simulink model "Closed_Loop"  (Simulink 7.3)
settings: Solver=ode45  StartTime=0.0  StopTime=10.0  RelTol=1e-3
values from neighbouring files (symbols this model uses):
  Acl = [    [closedloop.m]    (also in closedloop_eo.m)
  Bcl = [    [closedloop.m]    (also in closedloop_eo.m)
  Ccl = [    [closedloop.m]    (also in closedloop_eo.m)
  Dcl = [    [closedloop.m]    (also in closedloop_eo.m)

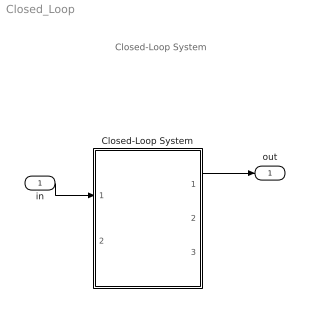
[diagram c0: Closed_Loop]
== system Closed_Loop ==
  note: Closed-Loop System
  in : Inport  OutDataType=sfix(16)  OutScaling=2^0
  Closed-Loop System : Subsystem
  out : Outport  OutDataType=sfix(16)  OutScaling=2^0
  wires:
  in/1 -> Closed-Loop System/1(atti)
  Closed-Loop System/1(attit) -> out/1

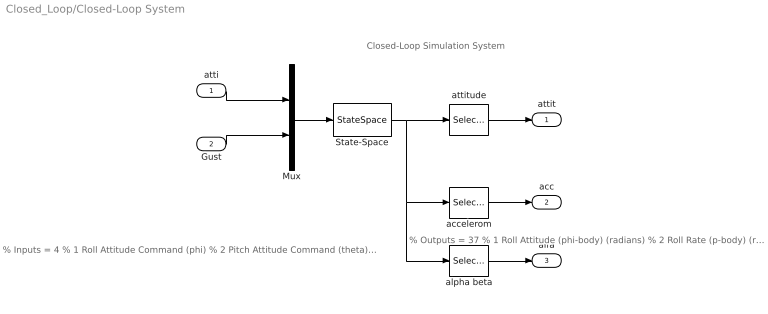
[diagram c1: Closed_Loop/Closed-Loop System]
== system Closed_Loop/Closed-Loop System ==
  note: % Inputs = 4 % 1 Roll Attitude Command (phi) % 2 Pitch Attitude Command (theta) % 3 Yaw Attitude Command (psi) % 4 Wind Gust Velocity (ft/sec)
  note: % Outputs = 37 % 1 Roll Attitude (phi-body) (radians) % 2 Roll Rate (p-body) (rad/sec) % 3 Pitch Attitude (thet-bdy) (radians) % 4 Pitch Rate (q-body) (rad/sec) % 5 Yaw Attitude (psi-body) (radians) % 6 Yaw Rate (r-body) (rad/sec) % 7 Angle of attack, alfa, (radians) % 8 Angle of sideslip, beta, (radian) % 9 Change in Altitude, delta-h, (feet) % 10 Forward Acceleration (V-dot) (ft/sec) % 11 Cross Range Velocity (Vcr) (ft/sec) % 12 Accelerom # 1, (along Z), (ft/sec^2) Translat. Acceler % 13 Accelerom # 2, (along Y), (ft/sec^2) Translat. Acceler % 14 Engine-1 Pitch Deftect (rad) % 15 Engine-2 Pitch Deftect (rad) % 16 Engine-3 Pitch Deftect (rad) % 17 Engine-4 Pitch Deftect (rad) % 18 Engine-5 Pitch Deftect (rad) % 19 Engine-6 Pitch Deftect (rad) % 20 Engine-7 Pitch Deftect (rad) % 21 Engine-8 Pitch Deftect (rad) % 22 Engine-9 Pitch Deftect (rad) % 23 Engine-1 Yaw Deftect (rad) % 24 Engine-2 Yaw Deftect (rad) % 25 Engine-3 Yaw Deftect (rad) % 26 Engine-4 Yaw Deftect (rad) % 27 Engine-5 Yaw Deftect (rad) % 28 Engine-6 Yaw Deftect (rad) % 29 Engine-7 Yaw Deftect (rad) % 30 Engine-8 Yaw Deftect (rad) % 31 Engine-9 Yaw Deftect (rad) % 32 Engine-4 Throttle % 33 Engine-5 Throttle % 34 Engine-6 Throttle % 35 Engine-7 Throttle % 36 Engine-8 Throttle % 37 Engine-9 Throttle
  note: Closed-Loop Simulation System
  atti : Inport  OutDataType=sfix(16)  OutScaling=2^0
  Gust : Inport  Port=2  OutDataType=sfix(16)  OutScaling=2^0
  Mux : Mux  Inputs=[3, 1]
  State-Space : StateSpace  A=Acl  B=Bcl  C=Ccl  D=Dcl
  accelerom : Selector  InputPortWidth=37  IndexOptions=Index vector (dialog)  Indices="[12,  13]"  OutputSizes=1
  alpha beta : Selector  InputPortWidth=37  IndexOptions=Index vector (dialog)  Indices="[7,  8]"  OutputSizes=1
  attitude : Selector  InputPortWidth=37  IndexOptions=Index vector (dialog)  Indices=[1, 3, 5]  OutputSizes=1
  attit : Outport  OutDataType=sfix(16)  OutScaling=2^0
  acc : Outport  Port=2  OutDataType=sfix(16)  OutScaling=2^0
  alfa : Outport  Port=3  OutDataType=sfix(16)  OutScaling=2^0
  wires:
  Mux/1 -> State-Space/1
  atti/1 -> Mux/1
  Gust/1 -> Mux/2
  State-Space/1 -> attitude/1, accelerom/1, alpha beta/1
  attitude/1 -> attit/1
  accelerom/1 -> acc/1
  alpha beta/1 -> alfa/1
